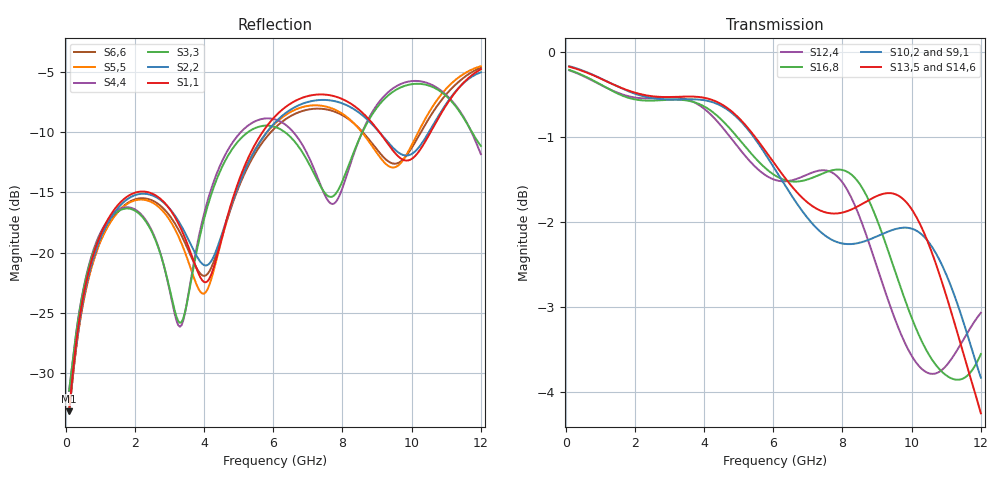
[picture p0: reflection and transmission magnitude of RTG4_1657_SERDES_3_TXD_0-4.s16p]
! RTG4 1657 S-parameter file
! Microsemi Corporation (c) 2019
!Initial ver: Jul 30, 2019
! Port::PIN_NAME::NET_NAME::S-parameter ports::PORT SIDE
! Port1:--:SERDES_3_TXD0_N_DIE::1::DIE
! Port2:--:SERDES_3_TXD0_P_DIE::2::DIE
! Port3:AU23:SERDES_3_TXD0_N_BGA::3::BGA
! Port4:AT23:SERDES_3_TXD0_P_BGA::4::BGA
! Port5:--:SERDES_3_TXD1_N_DIE::5::DIE
! Port6:--:SERDES_3_TXD1_P_DIE::6::DIE
! Port7:AW24:SERDES_3_TXD1_N_BGA::7::BGA
! Port8:AV24:SERDES_3_TXD1_P_BGA::8::BGA
! Port9:--:SERDES_3_TXD2_N_DIE::9::DIE
! Port10:--:SERDES_3_TXD2_P_DIE::10::DIE
! Port11:AU25:SERDES_3_TXD2_N_BGA::11::BGA
! Port12:AT25:SERDES_3_TXD2_P_BGA::12::BGA
! Port13:--:SERDES_3_TXD3_N_DIE::13::DIE
! Port14:--:SERDES_3_TXD3_P_DIE::14::DIE
! Port15:AU27:SERDES_3_TXD3_N_BGA::15::BGA
! Port16:AT27:SERDES_3_TXD3_P_BGA::16::BGA
!TouchstoneFormatFlag = 1
! GNDNET
! NETSLIST
! User Comments:
! Touchstone file exported from HFSS 2018.2.0
!  File:  //LSI_Z840_SIM_PC/Simulation_Data/MASUMISU/Microsemi_190710/YBD197_150320_NETCHANGE_SERDES_3_TXD.aedt
!  Generated:  8:56:09 ??  7 16, 2019
!  Design:  HFSSModel1
!  Project:  YBD197_150320_NETCHANGE_SERDES_3_TXD
!  Setup:  Setup1
!  Solution:  Sweep
! Terminal data exported
! Port[1] = SERDES_3_TXD0_N_DIE
! Port[2] = SERDES_3_TXD0_P_DIE
! Port[3] = SERDES_3_TXD1_N_DIE
! Port[4] = SERDES_3_TXD1_P_DIE
! Port[5] = SERDES_3_TXD2_N_DIE
! Port[6] = SERDES_3_TXD2_P_DIE
! Port[7] = SERDES_3_TXD3_N_DIE
! Port[8] = SERDES_3_TXD3_P_DIE
! Port[9] = SERDES_3_TXD0_N_BGA
! Port[10] = SERDES_3_TXD0_P_BGA
! Port[11] = SERDES_3_TXD1_N_BGA
! Port[12] = SERDES_3_TXD1_P_BGA
! Port[13] = SERDES_3_TXD2_N_BGA
! Port[14] = SERDES_3_TXD2_P_BGA
! Port[15] = SERDES_3_TXD3_N_BGA
! Port[16] = SERDES_3_TXD3_P_BGA
# GHZ S DB R 50.000000
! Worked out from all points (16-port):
!   239 points, 100 MHz to 12 GHz, reference 50 ohm
!   strongest paths, dB at 100 MHz, 3.05 GHz, 6.05 GHz, 9.05 GHz, 12 GHz:
!     S13,5: -0.2, -0.5, -1.3, -1.7, -4.3
!     S14,6: -0.2, -0.6, -1.4, -1.7, -3.9
!     S10,2: -0.2, -0.6, -1.4, -2.2, -3.8
!     S16,8: -0.2, -0.6, -1.5, -2.0, -3.6
!     S12,4: -0.2, -0.5, -1.5, -2.6, -3.1
!     S9,1: -0.2, -0.5, -1.4, -2.2, -3.8
!   lowest |S11| = -33.2 dB at 100 MHz (marker M1), VSWR 1.04, Z = 51.8 - j1.36 ohm
!   |S11| at or under -10 dB: start of sweep to 5.691 GHz; 9.065 GHz to 10.55 GHz (1.481 GHz wide, 15.1 % of centre)
